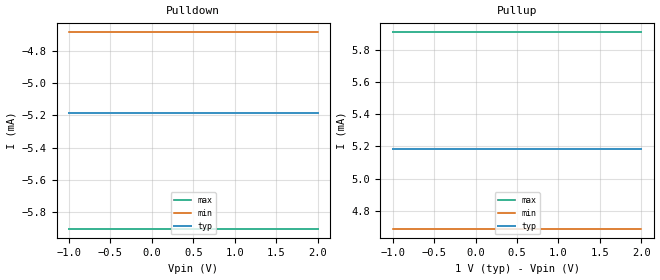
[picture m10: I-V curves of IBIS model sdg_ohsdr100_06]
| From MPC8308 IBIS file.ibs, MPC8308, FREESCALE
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[Model]   sdg_ohsdr100_06
Model_type 3-state
Enable Active-High
Polarity Non-Inverting
|   TYP   MIN   MAX
C_comp   0.00pF   0.00pF   0.00pF
[Model Spec]
Vmeas   0.5   0.45   0.55
[Temperature Range] 65   125   -40
[Voltage Range]   1.0   0.9   1.1
[Pullup]
|   Vout(V)   TYP   WCS   BCS
-1V       5.187mA    4.692mA    5.906mA
2V        5.187mA    4.692mA    5.906mA
[Pulldown]
|   Vout(V)   TYP   WCS   BCS
-1V       -5.187mA   -4.686mA   -5.902mA
2V        -5.187mA   -4.686mA   -5.902mA
[GND Clamp]
|   Vout(V)   TYP   WCS   BCS
-1V       0A         0A         0A
1V        0A         0A         0A
[POWER Clamp]
|   Vout(V)   TYP   WCS   BCS
-1V       0A         0A         0A
0V        0A         0A         0A
[Ramp]
R_load=50
dV/dt_r  3.0563e-01/2.7501e-11  2.7585e-01/3.2692e-11  3.3540e-01/3.3179e-11
dV/dt_f  3.0564e-01/3.3393e-11  2.7586e-01/3.5723e-11  3.3542e-01/3.7500e-11
|[End   sdg_ohsdr100_06
